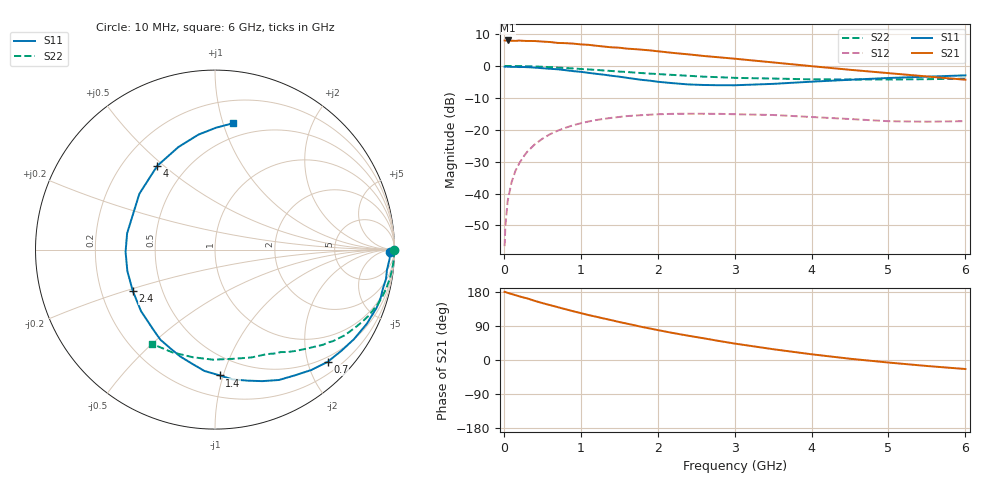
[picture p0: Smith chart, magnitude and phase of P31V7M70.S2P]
! SIEMENS Small Signal Semiconductors
! BFP181
! Si NPN RF Bipolar Junction Transistor in SOT143
! VCE = 1.75 V  IC = 0.7 mA
! Common Emitter S-Parameters:  March  1996
# GHz  S  MA  R  50
!  f  S11  S21  S12  S22
! GHz  MAG  ANG  MAG  ANG  MAG  ANG  MAG  ANG
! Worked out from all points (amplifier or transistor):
!   36 points, 10 MHz to 6 GHz, reference 50 ohm
!   highest |S21| = 8.0 dB at 50 MHz (marker M1)
!   |S21| within 3 dB of that: start of sweep to 1.845 GHz
!   unconditionally stable (mu >= 1): 3.476 GHz to end of sweep
!   at 250 MHz: K = 0.08, MSG = 18.3 dB, |S12| = -28.6 dB
!   at 1.4 GHz: K = 0.46, MSG = 11.0 dB, |S12| = -16.3 dB
!   at 6 GHz: K = 1.39, MAG = 2.8 dB, |S12| = -17.3 dB
!   S11 on the Smith chart (normalised r, x): 10 MHz: 60, -26; 700 MHz: 0.41, -2.36; 1.4 GHz: 0.35, -0.97; 2.4 GHz: 0.34, -0.21; 4 GHz: 0.35, +0.47; 6 GHz: 0.38, +1.08
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0.01  0.9724 -0.7  2.503 179.8  0.0015 89.0  0.9994 -0.2
0.02  0.975 -1.4  2.488 179.5  0.0031 88.3  0.9968 -0.6
0.05  0.9742 -3.0  2.507 177.1  0.0077 90.2  0.9984 -1.6
0.1  0.9649 -6.7  2.482 174.2  0.015 84.9  0.9972 -3.1
0.15  0.9667 -9.8  2.467 171.2  0.0226 83.3  0.9956 -4.6
0.25  0.9615 -16.3  2.473 165.2  0.037 79.0  0.9902 -7.8
0.4  0.9416 -26.0  2.457 156.2  0.0587 72.4  0.9796 -12.3
0.5  0.9211 -32.8  2.409 150.2  0.0722 67.7  0.97 -15.3
0.7  0.8861 -44.9  2.294 139.5  0.0967 59.5  0.9431 -21.0
0.9  0.8292 -57.8  2.239 128.7  0.1177 51.3  0.9134 -26.1
1.1  0.7789 -70.2  2.142 118.6  0.1347 44.1  0.8809 -31.0
1.4  0.7014 -87.9  1.957 105.1  0.1537 34.0  0.8328 -37.7
1.5  0.6786 -95.0  1.931 100.2  0.1587 31.4  0.8153 -39.4
1.8  0.6035 -114.4  1.794 87.0  0.1696 23.7  0.7722 -44.6
2.2  0.5365 -140.1  1.599 71.2  0.1777 14.2  0.7226 -51.3
2.4  0.5129 -153.2  1.518 64.0  0.1784 10.0  0.7008 -54.5
3  0.498 169.5  1.298 43.4  0.1751 -0.2  0.6503 -63.5
3.5  0.5237 143.6  1.135 28.5  0.1704 -6.2  0.6343 -71.3
4  0.5668 124.6  0.992 15.1  0.1584 -10.4  0.6168 -80.6
4.5  0.6069 109.6  0.87 3.3  0.1473 -13.0  0.6134 -91.0
5.5  0.6787 89.6  0.684 -15.8  0.1337 -9.2  0.6198 -112.6
6  0.7119 81.8  0.608 -23.8  0.1364 -6.2  0.6319 -123.8
